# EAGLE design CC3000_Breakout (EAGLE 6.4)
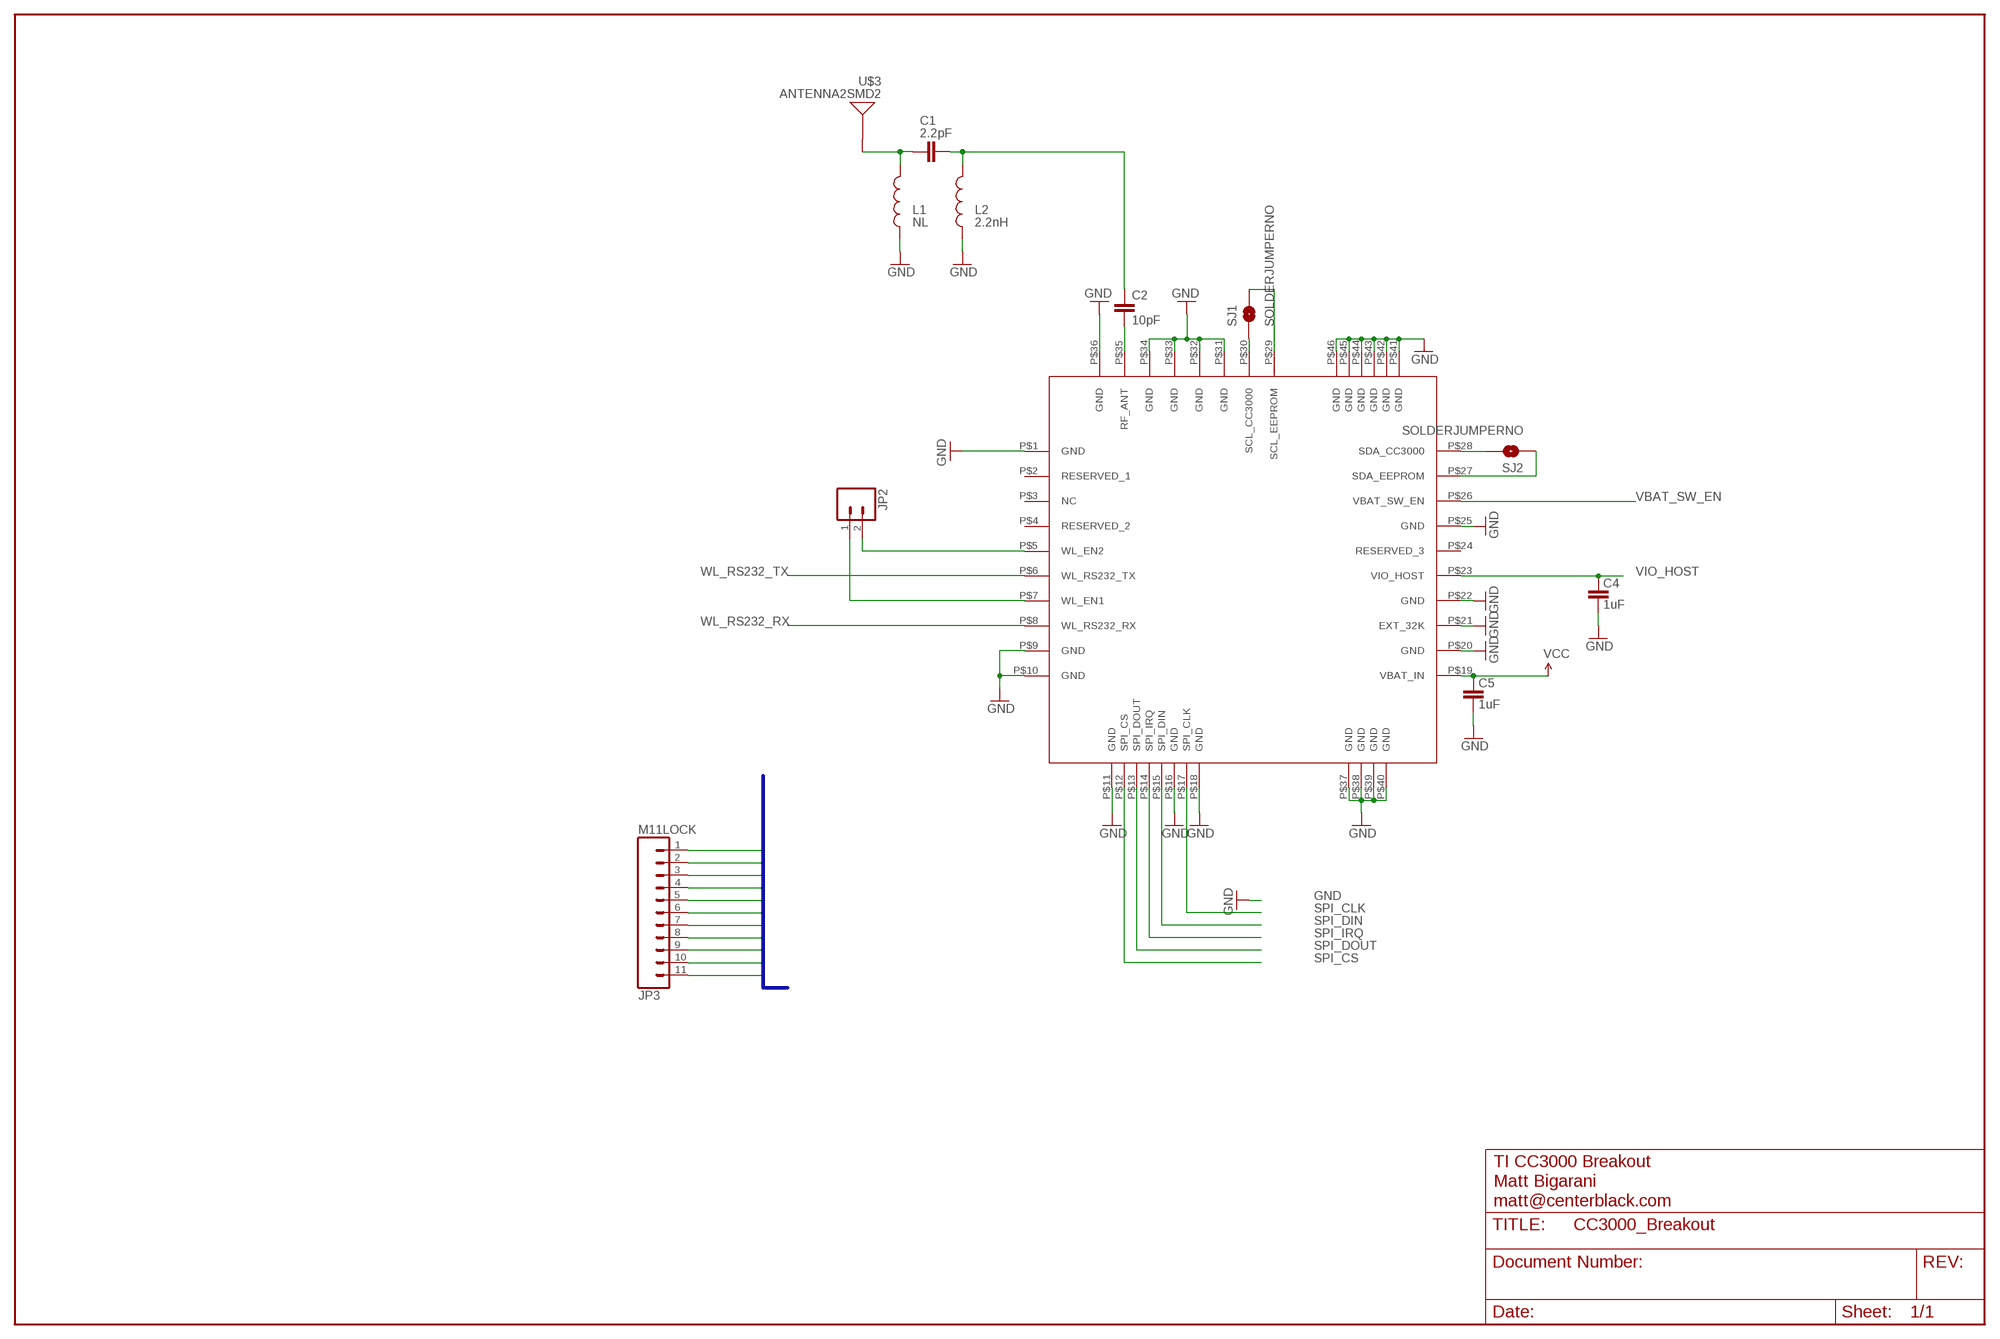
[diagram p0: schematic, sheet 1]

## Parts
C1  2.2pF  CAP0402-CAP  [0402-CAP]
C2  10pF  CAP0402-CAP  [0402-CAP]
C4  1uF  CAP0402-CAP  [0402-CAP]
C5  1uF  CAP0402-CAP  [0402-CAP]
JP2  M02LOCK  [1X02_LOCK]
JP3  M11LOCK  [1X11_LOCK]
L1  NL  INDUCTOR0402  [C0402]
L2  2.2nH  INDUCTOR0402  [C0402]
SJ1  SOLDERJUMPERNO  [SJ_2S-NO]
SJ2  SOLDERJUMPERNO  [SJ_2S-NO]
U$1  CC3000  [CC3000]
U$3  ANTENNA2SMD2  [ANTENNA-CHIP3]

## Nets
3.3V: C5.2 JP3.11 U$1.P$19(VBAT_IN) ; supply symbol labelled VCC
GND: C4.1 C5.1 JP3.10 L1.1 L2.1 U$1.P$1(GND) U$1.P$9(GND) U$1.P$10(GND) U$1.P$11(GND) U$1.P$16(GND) U$1.P$18(GND) U$1.P$20(GND) U$1.P$21(EXT_32K) U$1.P$22(GND) U$1.P$25(GND) U$1.P$31(GND) U$1.P$32(GND) U$1.P$33(GND) U$1.P$34(GND) U$1.P$36(GND) U$1.P$37(GND) U$1.P$38(GND) U$1.P$39(GND) U$1.P$40(GND) U$1.P$41(GND) U$1.P$42(GND) U$1.P$43(GND) U$1.P$44(GND) U$1.P$45(GND) U$1.P$46(GND)
N$10: C1.2 C2.1 L2.2
N$13: C2.2 U$1.P$35(RF_ANT)
N$14: SJ1.1 U$1.P$30(SCL_CC3000)
N$15: C1.1 L1.2 U$3.FEED(SIGNAL)
N$16: SJ1.2 U$1.P$29(SCL_EEPROM)
N$17: SJ2.2 U$1.P$28(SDA_CC3000)
N$18: SJ2.1 U$1.P$27(SDA_EEPROM)
SPI_CLK: JP3.7 U$1.P$17(SPI_CLK)
SPI_CS: JP3.3 U$1.P$12(SPI_CS)
SPI_DIN: JP3.6 U$1.P$15(SPI_DIN)
SPI_DOUT: JP3.4 U$1.P$13(SPI_DOUT)
SPI_IRQ: JP3.5 U$1.P$14(SPI_IRQ)
VBAT_SW_EN: JP3.9 U$1.P$26(VBAT_SW_EN)
VIO_HOST: C4.2 JP3.8 U$1.P$23(VIO_HOST)
WL_EN1: JP2.1 U$1.P$7(WL_EN1)
WL_EN2: JP2.2 U$1.P$5(WL_EN2)
WL_RS232_RX: JP3.2 U$1.P$8(WL_RS232_RX)
WL_RS232_TX: JP3.1 U$1.P$6(WL_RS232_TX)
Unconnected: U$1.P$2(RESERVED_1) U$1.P$3(NC) U$1.P$4(RESERVED_2) U$1.P$24(RESERVED_3)

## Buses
VBAT_SW_EN,VIO_HOST,SPI_CLK,SPI_DIN,SPI_IRQ,SPI_DOUT,SPI_CS,WL_RS232_RX,WL_RS232_TX,GND,VCC

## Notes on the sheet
- TI CC3000 Breakout
- Matt Bigarani
- matt@centerblack.com

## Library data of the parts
C1 C2 C4 C5 = SparkFun:CAP: Capacitor
JP2 = SparkFun:M02: Header 2
JP3 = SparkFun:M11: Header 11 Standard 11-pin 0.1" header. Use with straight break away headers (SKU : PRT-00116), right angle break away headers (PRT-00553), swiss pins (PRT-00743), machine pins (PRT-00117), and female headers (PRT-00115).
L1 L2 = SparkFun:INDUCTOR: Inductors
SJ1 SJ2 = SparkFun:SOLDERJUMPER: Solder Jumper
U$1 = centerblack_engineering:CC3000: TI SimpleLink CC3000 Module - WiFi 802.11b/g Network Processor; AUTHOR: Matt Bigarani; DATASHEET: http://www.ti.com/lit/ds/symlink/cc3000.pdf; DATE: 2/8/2013
U$3 = SparkFun:ANTENNA2: Antenna

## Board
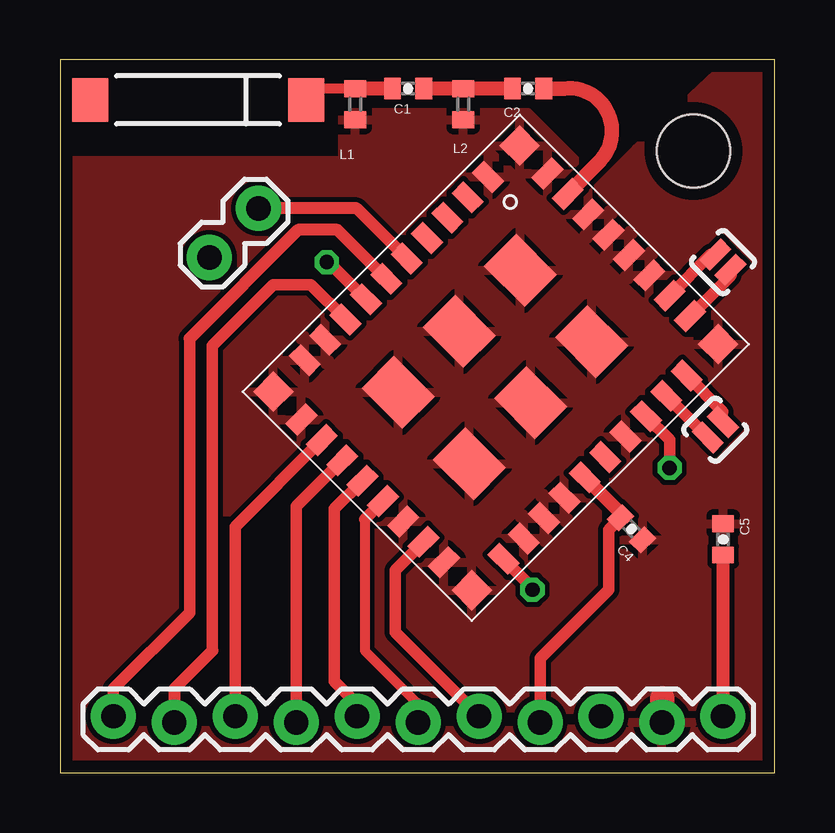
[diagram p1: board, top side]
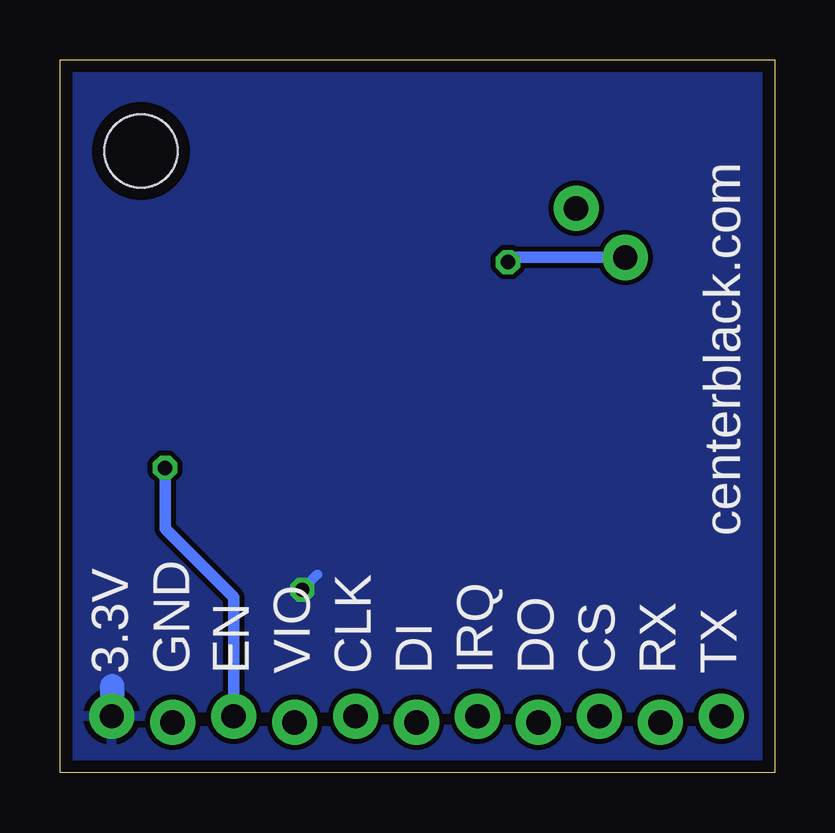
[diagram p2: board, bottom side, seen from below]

Size 29.78 x 29.69 mm. Coordinates in mm from the lower left corner, seen from the top.
Outline: 0,0 29.78,0 29.78,29.69 0,29.69 0,0
Copper layers (1*16): Top 0.035mm / dielectric 1.5mm / Bottom 0.035mm
Design rules "default *": minimum track width 10mil, minimum drill 24mil, track to track 8mil, track to pad 8mil, pad to pad 8mil, via to via 8mil, smd to smd 8mil, copper to edge 20mil, drill to drill 8mil, minimum pad ring 10mil, minimum via ring 8mil, stop-mask expansion 4mil, vias tented up to drill 0mil, thermal gap 10mil

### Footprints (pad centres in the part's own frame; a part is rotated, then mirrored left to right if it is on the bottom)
0402-CAP = smd 0.7 x 0.9: 1 -0.65,0; 2 0.65,0
1X02_LOCK = drill 1.016 pad 1.88: 1 -0.178,0; 2 2.718,0
1X11_LOCK = drill 1.016 pad 1.88: 1 0,0.127; 2 2.54,-0.127; 3 5.08,0.127; 4 7.62,-0.127; 5 10.16,0.127; 6 12.7,-0.127; 7 15.24,0.127; 8 17.78,-0.127; 9 20.32,0.127; 10 22.86,-0.127; 11 25.4,0.127
C0402 = smd 0.7 x 0.9: 1 -0.65,0; 2 0.65,0
SJ_2S-NO = smd 0.635 x 1.27: 1 -0.45,0; 2 0.45,0
CC3000 = smd 1.2 x 0.7: P$1 0.9,13.55; P$2 0.9,12.35; P$3 0.9,11.15; P$4 0.9,9.95; P$5 0.9,8.75; P$6 0.9,7.55; P$7 0.9,6.35; P$8 0.9,5.15; P$9 0.9,3.95; P$10 0.9,2.75; P$19 12.6,2.75; P$20 12.6,3.95; P$21 12.6,5.15; P$22 12.6,6.35; P$23 12.6,7.55; P$24 12.6,8.75; P$25 12.6,9.95; P$26 12.6,11.15; P$27 12.6,12.35; P$28 12.6,13.55 | smd 0.7 x 1.2: P$11 2.55,0.9; P$12 3.75,0.9; P$13 4.95,0.9; P$14 6.15,0.9; P$15 7.35,0.9; P$16 8.55,0.9; P$17 9.75,0.9; P$18 10.95,0.9; P$29 10.95,15.4; P$30 9.75,15.4; P$31 8.55,15.4; P$32 7.35,15.4; P$33 6.15,15.4; P$34 4.95,15.4; P$35 3.75,15.4; P$36 2.55,15.4 | smd 2.4 x 1.9: P$37 4.6,11.75; P$38 4.6,8.15; P$39 4.6,4.55; P$40 8.8,11.75; P$41 8.8,8.15; P$42 8.8,4.55 | smd 1.2 x 1.2: P$43 0.9,15.4; P$44 0.9,0.9; P$45 12.6,0.9; P$46 12.6,15.4
STAND-OFF-TIGHT = hole 3.048: 0,0
ANTENNA-CHIP3 = smd 1.8 x 1.5: FEED 0,4.5; NC 0,-4.5

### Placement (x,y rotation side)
C1  14.5,28.5 0 top
C2  19.5,28.5 0 top
C4  23.81,10.16 135 top
C5  27.63,9.72 270 top
JP2  6.35,21.59 45 top
JP3  2.22,2.22 0 top
L1  12.3,27.85 90 top
L2  16.8,27.85 90 top
SJ1  27.62,21.27 315 top
SJ2  27.3,14.29 45 top
U$1  7.62,15.88 315 top
U$2  [STAND-OFF-TIGHT]  26.4,25.9 0 top
U$3  5.75,28.03 270 top

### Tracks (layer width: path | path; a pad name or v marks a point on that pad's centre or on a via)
3.3V  (via drill 0.6)
  Top 0.406: 19.68,7.7 v19.68,7.62
  Top 0.483: U$1.P$19 19.68,7.7
  Top 0.55: C5.2 JP3.11
  Bottom 0.406: v19.68,7.62 19.05,8.26
  Bottom 1.016: 27.6,2.2 27.6,3.6
  pour Bottom: -1.27,-1.27 -1.27,31.02 31.56,31.02 31.56,-1.27
GND
  Top 1.016: 25.1,3.1 25.1,2.1
  pour Top: 0,0 30,0 30,29.75 28,29.75 24,26 21.25,23.25 20.75,23.25 20.25,23.75 20.25,24.25 21.5,25.5 19.5,27.5 11.75,27.5 11.75,25.5 0,25.5
N$10
  Top 0.584: C2.1 L2.2 C1.2
N$13
  Top 0.6: U$1.P$35 22.5,25.5 arc141 21,28.5 C2.2
N$14
  Top 0.483: 27.12,21.59 U$1.P$30
  Top 0.508: SJ1.1 27.12,21.59
N$15
  Top 0.406: L1.2 10.5,28.5 arc90 10.25,28.25 U$3.FEED
  Top 0.584: C1.1 L1.2
N$16
  Top 0.483: 27.94,20.71 U$1.P$29
  Top 0.508: SJ1.2 27.94,20.71
N$17
  Top 0.406: 27.62,15.03 SJ2.2
  Top 0.483: U$1.P$28 27.62,15.03
N$18
  Top 0.406: SJ2.1
  Top 0.483: U$1.P$27 SJ2.1
SPI_CLK
  Top 0.483: U$1.P$17 13.97,8.44 13.97,5.84 JP3.7
SPI_CS
  Top 0.483: U$1.P$12 7.3,10.25 JP3.3
SPI_DIN
  Top 0.406: 12.7,10.56 12.7,5.08 14.92,2.86
  Top 0.483: U$1.P$15 12.7,10.56 | JP3.6 14.92,2.86
SPI_DOUT
  Top 0.483: U$1.P$13 9.84,11.1 JP3.4
SPI_IRQ
  Top 0.483: U$1.P$14 11.43,10.99 11.43,3.81 12.38,2.86 JP3.5
VBAT_SW_EN  (via drill 0.6)
  Top 0.483: U$1.P$26 25.4,13.86 v25.4,12.7
  Bottom 0.483: v25.4,12.7 25.4,10.16 22.54,7.3 JP3.9
VIO_HOST
  Top 0.406: 23.35,10.82 C4.2
  Top 0.483: C4.2 22.86,10.13 22.86,7.62 20,4.76 JP3.8
  Top 0.559: U$1.P$23 23.35,10.82
WL_EN1  (via drill 0.6)
  Top 0.406: 11.2,21.27 v11.11,21.27
  Top 0.483: U$1.P$7 11.2,21.27
  Bottom 0.406: v11.11,21.27 10.92,21.46
  Bottom 0.483: 10.92,21.46 JP2.1
WL_EN2
  Top 0.483: U$1.P$5 12.36,23.51
  Top 0.5: 12.36,23.51 JP2.2
WL_RS232_RX
  Top 0.483: U$1.P$8 10.46,20.32 8.89,20.32 6.35,17.78 6.35,5.08
  Top 0.5: 6.35,5.08 4.76,3.49 JP3.2
WL_RS232_TX
  Top 0.483: U$1.P$6 11.56,22.61 | 5.4,18.1 5.4,6.67 2.22,3.49 JP3.1
  Top 0.5: 11.56,22.61 9.91,22.61 5.4,18.1

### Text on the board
bPlace: centerblack.com | TX | RX | CS | DO | IRQ | DI | CLK | VIO | EN | GND | 3.3V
